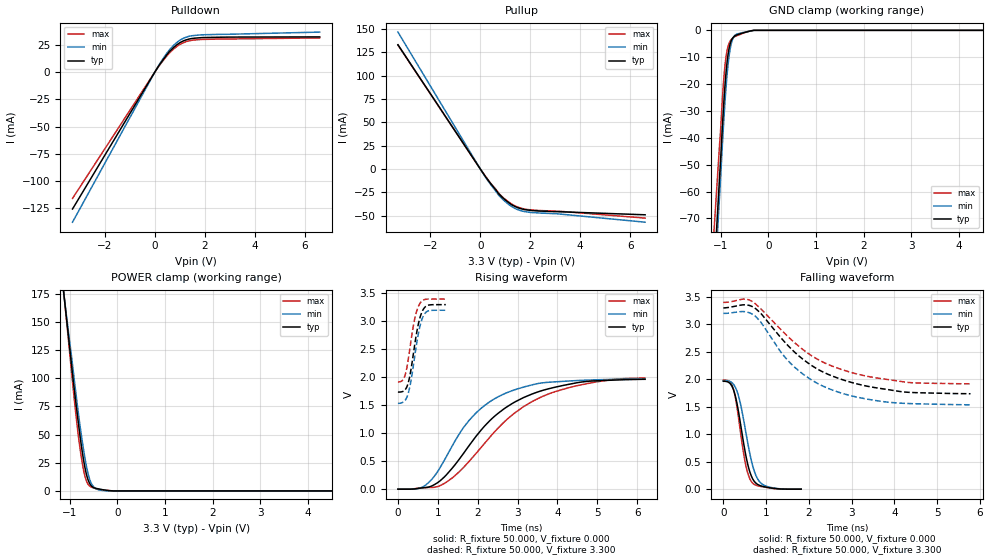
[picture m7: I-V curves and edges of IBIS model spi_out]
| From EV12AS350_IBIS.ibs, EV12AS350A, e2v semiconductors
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[Model]   spi_out
Model_type Output
Vref=0.000E+00
Rref=1.000E+06
Cref=0.000E+00
Vmeas=1.650E+00
C_comp   5.360E-13   5.110E-13   5.610E-13
[Voltage Range]   3.300E+00   3.200E+00   3.400E+00
[POWER Clamp Reference]   3.300E+00   3.200E+00   3.400E+00
[GND Clamp Reference]   0.000E+00   0.000E+00   0.000E+00
[Pullup Reference]   3.300E+00   3.200E+00   3.400E+00
[Pulldown Reference]   0.000E+00   0.000E+00   0.000E+00
[Temperature Range]   25   110   -40
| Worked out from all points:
|   slope of the pulldown table from 0 to 0.495 V, typ, clamps not added: 30.5 ohm
|   slope of the pullup table from 0 to 0.495 V, typ, clamps not added: 27.1 ohm
|   GND clamp passes 1 mA (typ) near -0.54 V on its own axis
|   POWER clamp passes 1 mA (typ) near -0.30 V on its own axis
|   rising waveform, R_fixture 50.000, V_fixture 0.000: 20-80 % time 1.59ns typ, 1.28ns min, 1.77ns max; typ from 0 V to 1.97 V
|   falling waveform, R_fixture 50.000, V_fixture 0.000: 20-80 % time 274ps typ, 305ps min, 237ps max; typ from 1.97 V to 0 V
|   rising waveform, R_fixture 50.000, V_fixture 3.300: 20-80 % time 219ps typ, 228ps min, 205ps max; typ from 1.74 V to 3.3 V
|   falling waveform, R_fixture 50.000, V_fixture 3.300: 20-80 % time 1.48ns typ, 1.33ns min, 1.54ns max; typ from 3.3 V to 1.74 V
[GND Clamp]
-3.3V     -764.7mA   -780.1mA   -672.3mA
-1.02V    -54.52mA   -61.43mA   -42.46mA
-1V       -48.68mA   -55.42mA   -37.57mA
-960mV    -35.41mA   -42.22mA   -25.2mA
-920mV    -23.81mA   -30.23mA   -15.53mA
-860mV    -11.39mA   -15.95mA   -7.237mA
-820mV    -6.643mA   -9.448mA   -4.789mA
-780mV    -4.074mA   -5.326mA   -3.537mA
-720mV    -2.346mA   -2.351mA   -2.555mA
-660mV    -1.706mA   -1.404mA   -2.034mA
-300mV    0A         0A         0A
6.6V      0A         0A         0A
[Power Clamp]
-3.3V     1.024A     927.9mA    1.118A
-1V       127.1mA    132.2mA    122.6mA
-920mV    95.97mA    104.5mA    87.98mA
-840mV    67.88mA    76.3mA     56.48mA
-740mV    35.67mA    45.09mA    25.79mA
-700mV    25.2mA     34.18mA    16.59mA
-640mV    13.26mA    20.08mA    7.916mA
-580mV    6.483mA    10.06mA    4.3mA
-540mV    4.177mA    6.046mA    3.287mA
-440mV    2.187mA    1.682mA    1.908mA
-180mV    332.6uA    18.18uA    245.9uA
6.6V      0A         0A         0A
[Pullup]
-3.3V     133mA      146.5mA    132.6mA
200mV     -7.849mA   -8.445mA   -7.51mA
720mV     -26.01mA   -27.52mA   -25.27mA
1.1V      -35.27mA   -37.19mA   -34.59mA
1.5V      -41.39mA   -43.48mA   -40.69mA
2.04V     -44.36mA   -46.52mA   -43.81mA
3.06V     -45.64mA   -47.85mA   -45.13mA
6.6V      -48.99mA   -56.9mA    -52.52mA
[Pulldown]
-3.3V     -125.6mA   -137.6mA   -115.9mA
60mV      2.199mA    2.403mA    2.044mA
500mV     16.39mA    17.84mA    15.23mA
760mV     22.58mA    24.55mA    21.2mA
900mV     25.23mA    27.33mA    23.68mA
1.08V     27.77mA    30.12mA    26.14mA
1.3V      29.68mA    32.22mA    28.13mA
1.76V     31.26mA    33.83mA    29.61mA
6.6V      32.11mA    36.51mA    31.17mA
[Rising Waveform]
R_fixture = 50.000
V_fixture = 0.000
V_fixture_min = 0.000
V_fixture_max = 0.000
|  time   V(typ)   V(min)   V(max)
0s        0V         0V         0V
660ps     26.92mV    55.63mV    26.99mV
920ps     83.23mV    237.2mV    34.02mV
1.2ns     244.8mV    563.5mV    118.2mV
1.78ns    774mV      1.226V     492.7mV
2.66ns    1.436V     1.703V     1.198V
3.18ns    1.647V     1.832V     1.489V
3.94ns    1.823V     1.919V     1.743V
5.1ns     1.942V     1.958V     1.932V
6.2ns     1.965V     1.976V     1.986V
[Falling Waveform]
R_fixture = 50.000
V_fixture = 0.000
V_fixture_min = 0.000
V_fixture_max = 0.000
|  time   V(typ)   V(min)   V(max)
0s        1.965V     1.976V     1.986V
200ps     1.876V     1.94V      1.898V
260ps     1.754V     1.883V     1.746V
320ps     1.555V     1.781V     1.487V
500ps     720.6mV    1.149V     532.4mV
580ps     421.7mV    802.4mV    268.6mV
660ps     229mV      504.8mV    133.6mV
780ps     97.93mV    218.3mV    65.89mV
940ps     46.87mV    76.09mV    40.48mV
1.82ns    0V         0V         0V
[Rising Waveform]
R_fixture = 50.000
V_fixture = 3.300
V_fixture_min = 3.200
V_fixture_max = 3.400
|  time   V(typ)   V(min)   V(max)
0s        1.737V     1.535V     1.917V
160ps     1.763V     1.573V     1.999V
200ps     1.797V     1.609V     2.091V
260ps     1.905V     1.717V     2.325V
320ps     2.109V     1.908V     2.619V
420ps     2.579V     2.371V     3.043V
540ps     3.035V     2.876V     3.308V
620ps     3.196V     3.07V      3.376V
720ps     3.279V     3.173V     3.398V
1.2ns     3.3V       3.2V       3.4V
[Falling Waveform]
R_fixture = 50.000
V_fixture = 3.300
V_fixture_min = 3.200
V_fixture_max = 3.400
|  time   V(typ)   V(min)   V(max)
0s        3.3V       3.2V       3.4V
500ps     3.356V     3.231V     3.461V
720ps     3.305V     3.165V     3.392V
1.36ns    2.744V     2.481V     2.893V
1.62ns    2.529V     2.254V     2.699V
2.08ns    2.243V     1.98V      2.421V
2.56ns    2.056V     1.802V     2.236V
3.3ns     1.885V     1.648V     2.065V
4.18ns    1.773V     1.564V     1.958V
5.78ns    1.737V     1.535V     1.917V
[Ramp]
dV/dt_r   1.1790E+00/1.5826E-09   1.1850E+00/1.2751E-09   1.1920E+00/1.7679E-09
dV/dt_f   9.3778E-01/1.4745E-09   9.9902E-01/1.3226E-09   8.8964E-01/1.5330E-09
R_load = 50
